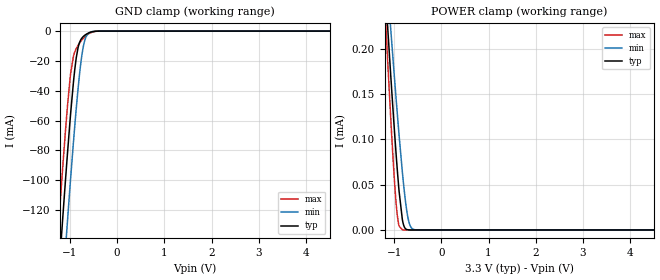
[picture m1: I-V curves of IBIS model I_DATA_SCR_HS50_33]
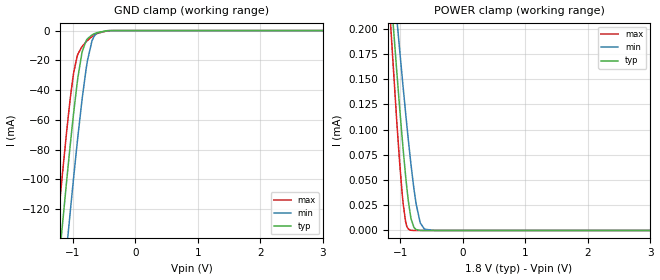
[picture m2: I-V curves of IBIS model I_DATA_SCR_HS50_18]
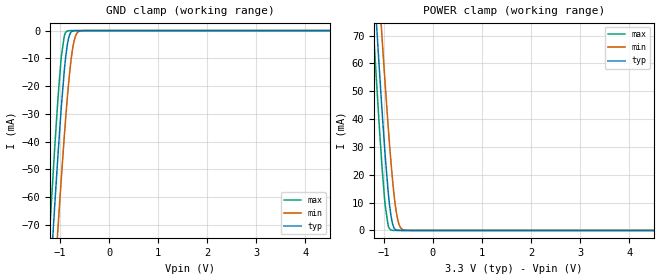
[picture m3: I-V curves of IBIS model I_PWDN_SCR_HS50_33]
| Texas Instruments Incorporated
| DS90UR908Q
| 5-65MHz 24-Bit Color FPD Link II to FPD-Link Converter
| Marketing part#   Voltage Range   Package-type   Temperature
| DS90UR908QSQE   1.71V - 3.6V   48-Pin LLP   -40 to 105C
| DS90UR908QSQ   1.71V - 3.6V   48-Pin LLP   -40 to 105C
| DS90UR908QSQX   1.71V - 3.6V   48-Pin LLP   -40 to 105C
[IBIS Ver]   4.0
[File name]   ds90ur908.ibs
[File Rev]   1.0
[Date]   03/27/2012
[Source]   Model built from TISPICE simulations at:
   Texas Instruments Incorporated.
   WEBENCH DESIGN CENTER
   12500 TI Blvd
   Dallas, TX -75243
   For Support e-mail: elab_scm_ibis@list.ti.com
[Notes]   Rev 1.0: 03/27/2012
   - Initial version of the IBIS model
   - All models are generated in Spectre
   - ccomp is listed in numerical order, for PVT information,
   please check notes above ccomp keyword for each model
   - All non-monotonic warnings can be ignored as per buffer behavior
[Disclaimer] This product is designed as an aid for customers of Texas Instruments.
   No warranties, either expressed or implied, with respect to this third
   party software (if any) or with respect to its fitness for any
   particular purpose is claimed by Texas Instruments or the author. The
   software (if any) is provided solely on an "as is" basis. The entire
   risk as to its quality and performance is with the customer
[Copyright]   (C)Copyright 2012 Texas Instruments Incorporated.
   All rights reserved.
|   DS90UR908Q
[Component]  DS90UR908Q
[Manufacturer]  Texas Instruments, Inc.
[Package]   |48 PIN llp
|   typ   min   max
R_pkg   0   0   0
L_pkg   0   0   0
C_pkg   0   0   0
[Pin]   signal_name   model_name   R_pin   L_pin   C_pin
1   PDB   I_PWDN_SCR_HS50
2   SSC[0]   IO_SMBUS_LVCMOS_HS50
3   SSC[1]   IO_SMBUS_LVCMOS_HS50
4   SDA   IO_SMBUS_LVCMOS_HS50
5   SCL   IO_SMBUS_LVCMOS_HS50
6   VDDL   POWER
7   SSC[2]   IO_DATA_50_HS50
8   VDDP   POWER
9   GND   GND
10   CONFIG[0]   IO_DATA_50_HS50
11   CONFIG[1]   IO_DATA_50_HS50
12   ID[x]   IO_DATA_50_HS50
13   VDDTX   POWER
14   GND   GND
15   TxOUT3+   NC
16   TxOUT3-   NC
17   TxCLKOUT+   NC
18   TxCLKOUT-   NC
19   TxOUT2+   NC
20   TxOUT2-   NC
21   TxOUT1+   NC
22   TxOUT1-   NC
23   TxOUT0+   NC
24   TxOUT0-   NC
25   VDDIO   POWER
26   GND   GND
27   LOCK   IO_DATA_50_ATP_HS50
28   PASS/EQ   IO_DATA_50_ATP_HS50
29   BISTEN   IO_DATA_50_HS50
30   OEN   IO_DATA_50_HS50
31   VDDL   POWER
32   GND   GND
33   VODSEL   IO_DATA_50_HS50
34   MAPSEL   IO_DATA_50_HS50
35   OSS_SEL   IO_DATA_50_HS50
36   LFMODE   IO_DATA_50_HS50
37   RES   NC
38   VDDA   POWER
39   GND   GND
40   RIN+   NC
41   RIN-   NC
42   CMF   NC
43   VDDA   POWER
44   GND   GND
45   GND   GND
46   VDDSC   POWER
47   VDDSC   POWER
48   GND   GND
49   DAP   GND
[Package Model]  llp48_ds90ur908QSQ
[Diff pin]  inv_pin  vdiff  tdelay_typ  tdelay_min  tdelay_max
15   16   0.0   0.0s   0.0s   0.0s
17   18   0.0   0.0s   0.0s   0.0s
19   20   0.0   0.0s   0.0s   0.0s
21   22   0.0   0.0s   0.0s   0.0s
23   24   0.0   0.0s   0.0s   0.0s
[Model Selector]   I_DATA_SCR_HS50
I_DATA_SCR_HS50_33   I_DATA_SCR_HS50 input with VDD=3.3V
I_DATA_SCR_HS50_18   I_DATA_SCR_HS50 input with VDD=1.8V
[Model Selector]   I_DATA_MC_HS50
I_DATA_MC_HS50_33   I_DATA_MC_HS50 input with VDD=3.3V
I_DATA_MC_HS50_18   I_DATA_MC_HS50 input with VDD=1.8V
[Model Selector]   I_PWDN_SCR_HS50
I_PWDN_SCR_HS50_33   I_PWDN_SCR_HS50 input with VDD=3.3V
I_PWDN_SCR_HS50_18   I_PWDN_SCR_HS50 input with VDD=1.8V
[Model Selector]   IO_DATA_50_HS50
IO_DATA_50_HS50_33   IO_DATA_50_HS50 with VDD=3.3V
IO_DATA_50_HS50_18   IO_DATA_50_HS50 with VDD=1.8V
[Model Selector]   IO_DATA_50_ATP_HS50
IO_DATA_50_ATP_HS50_33   IO_DATA_50_ATP_HS50 with VDD=3.3V
IO_DATA_50_ATP_HS50_18   IO_DATA_50_ATP_HS50 with VDD=1.8V
[Model Selector]   IO_SMBUS_HS50
IO_SMBUS_HS50_33   IO_SMBUS_HS50 with VDD=3.3V
IO_SMBUS_HS50_18   IO_SMBUS_HS50 with VDD=1.8V
[Model Selector]   IO_SMBUS_LVCMOS_HS50
IO_SMBUS_LVCMOS_HS50_33_HI   IO_SMBUS_HS50 HI DRIVE with VDD=3.3V
IO_SMBUS_LVCMOS_HS50_33_LO   IO_SMBUS_HS50 LO DRIVE with VDD=3.3V
IO_SMBUS_LVCMOS_HS50_18_HI   IO_SMBUS_HS50 HI DRIVE with VDD=1.8V
IO_SMBUS_LVCMOS_HS50_18_LO   IO_SMBUS_HS50 LO DRIVE with VDD=1.8V
|   DS90UR908Q   Package model
[Define Package Model]  llp48_ds90ur908QSQ
[Manufacturer]  Texas Instruments, Inc
[OEM]  Texas Instruments, Inc
[Description]  Package leads with wirebonds at 3GHz
[Number Of Pins]  49
[Pin Numbers]
49   | 49 = DAP
1   | 1 = L1
2   | 2 = L2
3   | 3 = L3
4   | 4 = L4
5   | 5 = L5
6   | 6 = L6
7   | 7 = L7
8   | 8 = L8
9   | 9 = L9
10   | 10 = L10
11   | 11 = L11
12   | 12 = L12
13   | 13 = L13
14   | 14 = L14
15   | 15 = L15
16   | 16 = L16
17   | 17 = L17
18   | 18 = L18
19   | 19 = L19
20   | 20 = L20
21   | 21 = L21
22   | 22 = L22
23   | 23 = L23
24   | 24 = L24
25   | 25 = L25
26   | 26 = L26
27   | 27 = L27
28   | 28 = L28
29   | 29 = L29
30   | 30 = L30
31   | 31 = L31
32   | 32 = L32
33   | 33 = L33
34   | 34 = L34
35   | 35 = L35
36   | 36 = L36
37   | 37 = L37
38   | 38 = L38
39   | 39 = L39
40   | 40 = L40
41   | 41 = L41
42   | 42 = L42
43   | 43 = L43
44   | 44 = L44
45   | 45 = L45
46   | 46 = L46
47   | 47 = L47
48   | 48 = L48
[Model Data]
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[End Model Data]
[End Package Model]
| Models and submodels in the file (16): I_DATA_SCR_HS50_33 (Input), I_DATA_SCR_HS50_18 (Input), I_PWDN_SCR_HS50_33 (Input), I_PWDN_SCR_HS50_18 (Input), I_DATA_MC_HS50_18 (Input), I_DATA_MC_HS50_33 (Input), IO_SMBUS_HS50_33 (I/O_open_drain), IO_SMBUS_HS50_18 (I/O_open_drain), IO_DATA_50_HS50_33 (I/O), IO_DATA_50_HS50_18 (I/O), IO_DATA_50_ATP_HS50_33 (I/O), IO_DATA_50_ATP_HS50_18 (I/O), IO_SMBUS_LVCMOS_HS50_33_HI (I/O), IO_SMBUS_LVCMOS_HS50_33_LO (I/O), IO_SMBUS_LVCMOS_HS50_18_HI (I/O), IO_SMBUS_LVCMOS_HS50_18_LO (I/O)
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|   Model I_DATA_SCR_HS50_33
[Model] I_DATA_SCR_HS50_33
Model_type Input
Vinl =   0.8
Vinh =   2.0
|   typ   min   max
|   (nom)   (slow)   (fast)
C_comp   0.3665pF   0.3665pF   0.3665pF
[Temperature Range]   25.000   105.000   -40.000
[Voltage Range]   3.300V   3.0000V   3.6000V
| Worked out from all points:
|   GND clamp passes 1 mA (typ) near -0.58 V on its own axis
|   POWER clamp passes 1 mA (typ) near -2.02 V on its own axis
[GND Clamp]
|   Voltage   I(typ)   I(min)   I(max)
-3.3V     -1.166A    -1.209A    -1.134A
-1.32V    -202.1mA   -249mA     -167.1mA
-1.241V   -165.6mA   -212.4mA   -130.7mA
-1.142V   -121mA     -167.4mA   -86.89mA
-1.063V   -86.78mA   -132.3mA   -54.56mA
-983.4mV  -54.93mA   -98.36mA   -28.27mA
-924mV    -33.98mA   -74.16mA   -16.74mA
-825mV    -10.8mA    -38mA      -9.446mA
-755.7mV  -5.134mA   -18.34mA   -6.356mA
-696.3mV  -3.098mA   -7.601mA   -4.22mA
-567.6mV  -815.5uA   -746uA     -1.217mA
6.59V     0A         0A         0A
[POWER Clamp]
|   Voltage   I(typ)   I(min)   I(max)
-3.3V     2.159mA    1.892mA    2.559mA
-1.191V   270.3uA    306.6uA    243.1uA
-1.132V   220.6uA    264.4uA    182.9uA
-1.063V   164.1uA    216.1uA    115.7uA
-993.3mV  110.2uA    168.9uA    55.28uA
-933.9mV  67.72uA    129.8uA    16.89uA
-894.3mV  42.8uA     104.8uA    4.336uA
-825mV    11.61uA    64.2uA     166.8nA
-755.7mV  1.271uA    30.48uA    2.122nA
-696.3mV  130.3nA    11.15uA    0A
-557.7mV  0A         260.4nA    0A
6.59V     0A         0A         0A
|   Model I_DATA_SCR_HS50_18
[Model] I_DATA_SCR_HS50_18
Model_type Input
Vinl =   0.63
Vinh =   1.17
|   typ   min   max
|   (nom)   (fast)   (slow)
C_comp   0.5298pF   0.3665pF   0.5298pF
[Temperature Range]   25.000   105.000   -40.000
[Voltage Range]   1.800V   1.7100V   1.8900V
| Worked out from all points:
|   GND clamp passes 1 mA (typ) near -0.56 V on its own axis
[GND Clamp]
|   Voltage   I(typ)   I(min)   I(max)
-1.8V     -430.9mA   -477mA     -396.6mA
-1.238V   -164.5mA   -211.3mA   -129.6mA
-1.174V   -135.2mA   -181.7mA   -100.7mA
-1.093V   -99.54mA   -145.4mA   -66.37mA
-1.039V   -76.81mA   -121.8mA   -45.69mA
-984.6mV  -55.39mA   -98.86mA   -28.59mA
-930.6mV  -36.12mA   -76.78mA   -17.61mA
-855mV    -15.77mA   -48.21mA   -11.06mA
-763.2mV  -5.498mA   -20.14mA   -6.658mA
-687.6mV  -2.877mA   -6.556mA   -3.945mA
-450mV    -97.64uA   -77.9uA    -176.8uA
3.595V    0A         0A         0A
[POWER Clamp]
|   Voltage   I(typ)   I(min)   I(max)
-1.8V     803.7uA    754.7uA    897.4uA
-1.157V   241.8uA    282.5uA    208.5uA
-1.055V   157.9uA    210.7uA    108.4uA
-1.012V   124.1uA    181.2uA    70.17uA
-952.2mV  80.3uA     141.7uA    26.6uA
-914.4mV  55uA       117.4uA    9.25uA
-865.8mV  27.6uA     87.52uA    1.228uA
-822.6mV  10.92uA    62.89uA    149.1nA
-747mV    921.8nA    26.99uA    1.513nA
-682.2mV  75.41nA    8.215uA    0A
-612mV    3.441nA    1.296uA    0A
3.595V    0A         0A         0A
|   Model I_PWDN_SCR_HS50_33
[Model] I_PWDN_SCR_HS50_33
Model_type Input
Vinl =   0.8
Vinh =   2.0
|   typ   min   max
|   (nom)   (fast)   (slow)
C_comp   0.3665pF   0.3665pF   0.5298pF
[Temperature Range]   25.000   105.000   -40.000
[Voltage Range]   3.300V   3.0000V   3.6000V
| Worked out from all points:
|   GND clamp passes 1 mA (typ) near -0.79 V on its own axis
|   POWER clamp passes 1 mA (typ) near -0.79 V on its own axis
[GND Clamp]
|   Voltage   I(typ)   I(min)   I(max)
-3.3V     -740.6mA   -745.8mA   -738.2mA
-1.211V   -92.27mA   -118mA     -71.83mA
-1.191V   -86.5mA    -112.3mA   -65.95mA
-1.112V   -63.85mA   -90.11mA   -43.04mA
-1.043V   -44.84mA   -71.14mA   -24.45mA
-973.5mV  -27.25mA   -52.87mA   -9.257mA
-914.1mV  -14.38mA   -38.09mA   -1.938mA
-854.7mV  -5.279mA   -24.66mA   -158.3uA
-785.4mV  -769.6uA   -11.9mA    -11.81uA
-726mV    -91.41uA   -4.691mA   -6.467uA
-577.5mV  -3.449uA   -99.25uA   -4.919uA
6.59V     0A         0A         0A
[POWER Clamp]
|   Voltage   I(typ)   I(min)   I(max)
-3.3V     739mA      744.2mA    736.5mA
-1.211V   92.02mA    117.6mA    71.62mA
-1.191V   86.27mA    112mA      65.75mA
-1.112V   63.66mA    89.86mA    42.89mA
-1.043V   44.7mA     70.93mA    24.36mA
-973.5mV  27.14mA    52.7mA     9.21mA
-914.1mV  14.31mA    37.95mA    1.931mA
-854.7mV  5.248mA    24.55mA    164.4uA
-785.4mV  767.3uA    11.83mA    19.72uA
-726mV    94.5uA     4.66mA     14.93uA
-577.5mV  8.162uA    100.4uA    14.65uA
6.59V     0A         0A         0A
